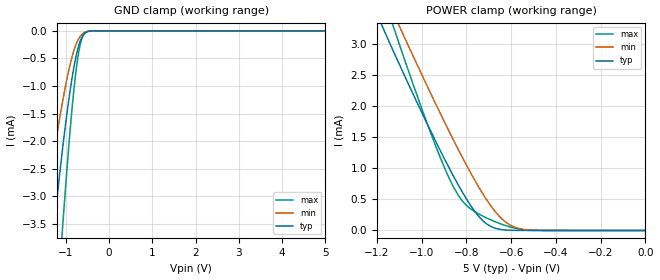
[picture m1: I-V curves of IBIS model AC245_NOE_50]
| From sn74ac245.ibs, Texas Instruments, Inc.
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[Model]   AC245_NOE_50
Model_type  Input
Vinl=1.35
Vinh=3.85
| variable   typ   min   max
C_comp   0.89pF   0.79pF   1.41pF
[Temperature Range]   40   100   -40
| Ambient temperature   25   85   -40
[Voltage range]   5   4.5   5.5
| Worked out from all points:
|   GND clamp passes 1 mA (typ) near -0.88 V on its own axis
|   POWER clamp passes 1 mA (typ) near -0.88 V on its own axis
[GND Clamp]
| AC245_NOE_50
|   Voltage   I(typ)   I(min)   I(max)
-5V       -46.92mA   -30.58mA   -59.62mA
-1.56V    -6.035mA   -3.826mA   -9.528mA
-1.51V    -5.59mA    -3.537mA   -8.882mA
-1.305V   -3.869mA   -2.418mA   -6.312mA
-1.255V   -3.478mA   -2.163mA   -5.708mA
-1.08V    -2.21mA    -1.334mA   -3.692mA
-1.06V    -2.076mA   -1.247mA   -3.474mA
-900mV    -1.111mA   -628.4uA   -1.852mA
-770mV    -508.4uA   -270.1uA   -799.3uA
-670mV    -203.9uA   -108.8uA   -280.1uA
-550mV    -38.99uA   -24.34uA   -40.29uA
5V        16.38nA    4.859uA    150.6nA
[POWER Clamp]
| AC245_NOE_50
|   Voltage   I(typ)   I(min)   I(max)
-5V       45.74mA    45.24mA    49.64mA
-1.17V    3.235mA    3.838mA    3.746mA
-1.125V   2.87mA     3.482mA    3.262mA
-1.075V   2.477mA    3.09mA     2.732mA
-965mV    1.638mA    2.244mA    1.62mA
-895mV    1.129mA    1.722mA    985.3uA
-840mV    755.6uA    1.327mA    587.5uA
-785mV    423.6uA    951.8uA    357.6uA
-695mV    72.53uA    417uA      176.8uA
-640mV    12.79uA    181.6uA    97.2uA
-585mV    1.851uA    53.91uA    37.94uA
-84.45fV  16.38nA    947.5pA    229.7nA
